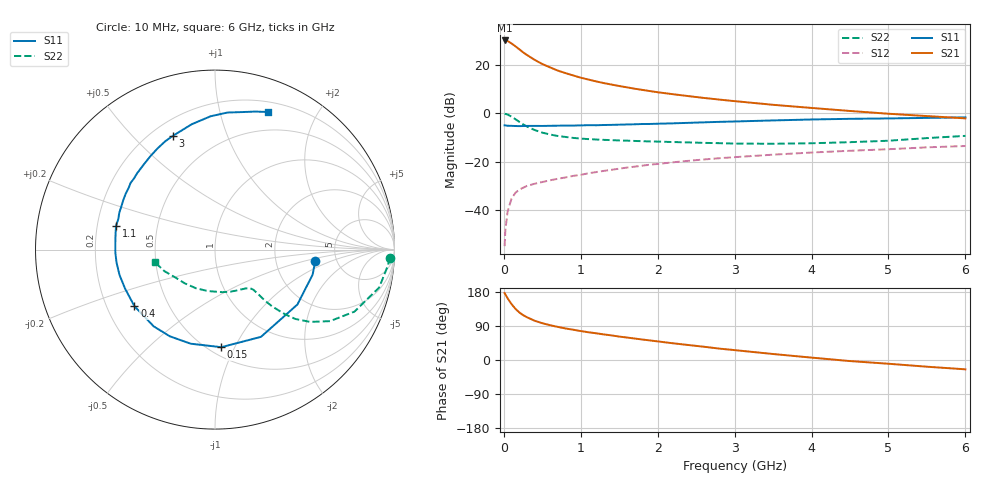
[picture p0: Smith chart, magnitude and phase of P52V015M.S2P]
! SIEMENS Small Signal Semiconductors
! BFP183
! Si NPN RF Bipolar Junction Transistor in SOT143
! VCE = 2 V  IC = 15 mA
! Common Emitter S-Parameters:  March  1996
# GHz  S  MA  R  50
!  f  S11  S21  S12  S22
! GHz  MAG  ANG  MAG  ANG  MAG  ANG  MAG  ANG
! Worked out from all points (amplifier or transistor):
!   36 points, 10 MHz to 6 GHz, reference 50 ohm
!   highest |S21| = 30.1 dB at 10 MHz (marker M1)
!   |S21| within 3 dB of that: start of sweep to 174.5 MHz
!   unconditionally stable (mu >= 1): 902.5 MHz to 5.579 GHz
!   at 250 MHz: K = 0.43, MSG = 28.0 dB, |S12| = -30.8 dB
!   at 1.4 GHz: K = 1.14, MAG = 15.3 dB, |S12| = -23.4 dB
!   at 6 GHz: K = 0.95, MSG = 5.7 dB, |S12| = -13.5 dB
!   S11 on the Smith chart (normalised r, x): 10 MHz: 3.43, -0.66; 150 MHz: 0.57, -0.89; 400 MHz: 0.32, -0.29; 1.1 GHz: 0.28, +0.11; 3 GHz: 0.28, +0.66; 6 GHz: 0.30, +1.42
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0.01  0.5619 -6.7  31.82 176.5  0.0018 83.6  0.9746 -2.6
0.02  0.5616 -14.4  31.81 173.2  0.0039 84.3  0.9679 -5.2
0.05  0.5517 -33.7  30.93 162.5  0.0095 79.8  0.9388 -13.0
0.1  0.5495 -62.2  27.57 147.5  0.0173 64.2  0.8502 -24.0
0.15  0.5449 -86.3  24.13 135.2  0.0227 58.1  0.7544 -31.9
0.2  0.5415 -104.5  20.96 125.7  0.0265 52.9  0.6646 -37.3
0.25  0.5447 -117.5  18.11 118.5  0.0289 49.2  0.5913 -40.8
0.3  0.5473 -128.6  15.97 112.9  0.0316 47.4  0.5326 -42.7
0.4  0.5486 -144.9  12.66 103.6  0.035 46.2  0.4503 -44.8
0.5  0.5462 -156.7  10.37 97.1  0.038 45.0  0.3979 -45.6
0.6  0.5504 -165.1  8.854 91.9  0.0412 46.1  0.3637 -45.8
0.7  0.5533 -172.4  7.606 87.4  0.0443 46.9  0.3396 -45.9
0.9  0.5566 176.2  6.034 80.0  0.0508 48.3  0.3098 -46.3
1.1  0.5671 166.5  4.955 73.2  0.0576 49.5  0.2921 -47.7
1.5  0.5807 151.7  3.646 61.8  0.0718 49.6  0.2743 -52.1
1.8  0.599 141.8  3.034 54.0  0.0827 48.7  0.2642 -57.1
2.2  0.6187 129.8  2.468 44.1  0.0971 46.5  0.2542 -65.0
3  0.6756 110.4  1.778 26.1  0.1239 40.7  0.2365 -85.3
3.5  0.7104 100.5  1.493 15.8  0.1396 36.7  0.2344 -100.1
4.5  0.7668 84.8  1.114 -2.8  0.1678 28.2  0.2526 -132.0
5.5  0.8012 73.7  0.874 -17.7  0.1977 20.6  0.3067 -157.0
6  0.8223 68.8  0.784 -24.6  0.2103 16.0  0.3409 -167.9
